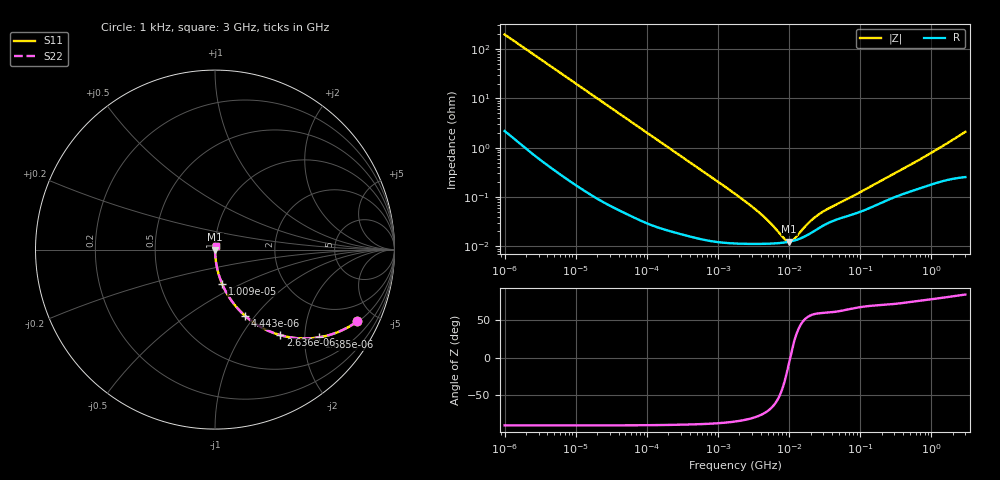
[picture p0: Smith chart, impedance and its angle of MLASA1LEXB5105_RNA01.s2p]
! MLASA1LEXB5105_RNA01  S-PARAMETER MODEL  ( Standard Model )
! Model Generated by TAIYO YUDEN Corporation (http://www.ty-top.com)
! Version 1.0
! TAIYO YUDEN Control No. 220601
! Copyright(c) 2015 TAIYO YUDEN CO.,LTD. All Rights Reserved.
! Product Description (link to TY-COMPAS)
! https://ds.yuden.co.jp/TYCOMPAS/or/detail?pn=MLASA1LEXB5105MRNA01&u=M
! Products Name : Multilayer Ceramic Capacitors
! Characteristics :
!  Capacitance : 1 [uF] , Rated Voltage : 4 [V] , TCC : X5R
!  Case Size : 1.0 x 0.5 / 0.039 x 0.02 [mm/inch] , Thickness : 0.18 / 0.007 [mm/inch]
!  (Conditions: Temperature = 25 [degC] , DC Bias Voltage = 0 [V])
! External Node Assignments :
!  1  o---| |---o  2
! GND o---------o GND
! Frequency Range : 1kHz  -  3GHz  [ 401 STEP ]
# MHZ S RI R 50
! Freq[MHz].  S11 Real  S11 Imag  S21 Real  S21 Imag  S12 Real  S12 Imag  S22 Real  S22 Imag
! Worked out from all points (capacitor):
!   401 points, 1 kHz to 3 GHz, reference 50 ohm
!   read as one part in series: C = 805 nF near 1.077 kHz
!   lowest |Z| = 12.5 mohm at 9.991 MHz (marker M1)
!   series resonance near 10.34 MHz, so ESL is about 290 pH
!   S11 on the Smith chart (normalised r, x): 1 kHz: 1.04, -3.95; 1.685 kHz: 1.02, -2.35; 2.636 kHz: 1.01, -1.51; 4.443 kHz: 1.01, -0.90; 10.09 kHz: 1.00, -0.40; 3 GHz: 1.01, +0.04
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0.001  0.7931 -0.3996  0.2069 0.3996  0.2069 0.3996  0.7931 -0.3996
0.001251  0.7121 -0.4475  0.2879 0.4475  0.2879 0.4475  0.7121 -0.4475
0.001685  0.5794 -0.4887  0.4206 0.4887  0.4206 0.4887  0.5794 -0.4887
0.002636  0.3633 -0.4764  0.6367 0.4764  0.6367 0.4764  0.3633 -0.4764
0.004443  0.1694 -0.3708  0.8306 0.3708  0.8306 0.3708  0.1694 -0.3708
0.006451  0.0893 -0.2809  0.9107 0.2809  0.9107 0.2809  0.0893 -0.2809
0.010091  0.0393 -0.19  0.9607 0.19  0.9607 0.19  0.0393 -0.19
0.01216  0.0277 -0.1598  0.9723 0.1598  0.9723 0.1598  0.0277 -0.1598
0.033275  0.00425 -0.0601  0.9957 0.0601  0.9957 0.0601  0.00425 -0.0601
0.147855  0.000425 -0.0137  0.9996 0.0137  0.9996 0.0137  0.000425 -0.0137
1.732051  0.000115 -0.00115  0.9999 0.00115  0.9999 0.00115  0.000115 -0.00115
3.93371  0.000112 -0.000448  0.9999 0.000448  0.9999 0.000448  0.000112 -0.000448
5.502215  0.000113 -0.000269  0.9999 0.000269  0.9999 0.000269  0.000113 -0.000269
8.606987  0.00012 -7.4e-05  0.9999 7.4e-05  0.9999 7.4e-05  0.00012 -7.4e-05
9.991309  0.000124 -1.39e-05  0.9999 1.39e-05  0.9999 1.39e-05  0.000124 -1.39e-05
10.76485  0.000127 1.6e-05  0.9999 -1.6e-05  0.9999 -1.6e-05  0.000127 1.6e-05
12.03889  0.000132 6.08e-05  0.9999 -6.08e-05  0.9999 -6.08e-05  0.000132 6.08e-05
21.06097  0.000193 0.000291  0.9998 -0.000291  0.9998 -0.000291  0.000193 0.000291
32.94519  0.000282 0.00047  0.9997 -0.00047  0.9997 -0.00047  0.000282 0.00047
256.0921  0.000902 0.00247  0.9991 -0.00247  0.9991 -0.00247  0.000902 0.00247
727.4359  0.00157 0.00582  0.9984 -0.00582  0.9984 -0.00582  0.00157 0.00582
3000  0.00296 0.0207  0.997 -0.0207  0.997 -0.0207  0.00296 0.0207
